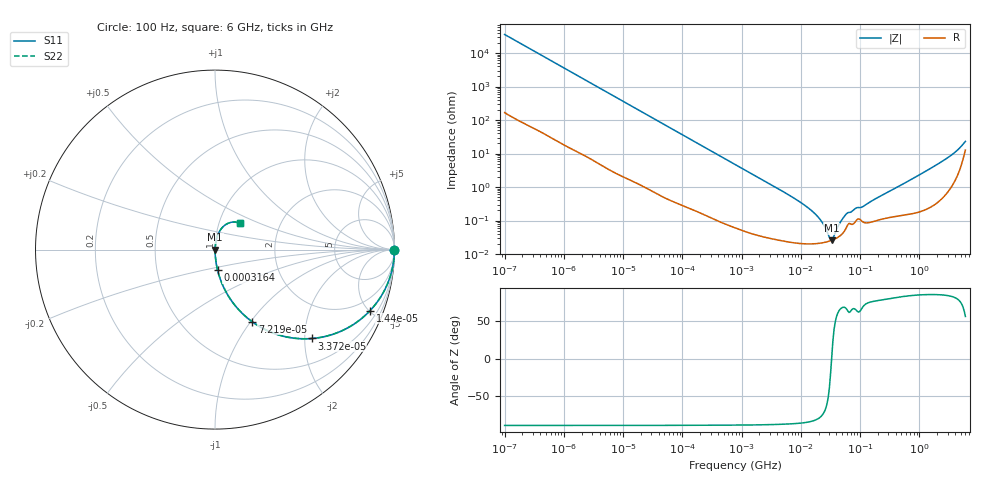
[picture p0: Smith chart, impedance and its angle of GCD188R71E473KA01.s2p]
!Murata Part Number: GCD188R71E473KA01
!These Parameters are Measured in Series Mode Connection
!Data Generated on Jan 08, 2026
!  o--ll--o
!Port1  Port2
!  o------o
!Operation Temp=25[degC], DC Bias Voltage=0[V]
!Freq. Start=100[Hz] Stop=6[GHz] 401[Steps]
# Hz S RI R 50
!Freq.(Hz) S11(Real) S11(Imag) S21(Real) S21(Imag) S12(Real) S12(Imag) S22(Real) S22(Imag)
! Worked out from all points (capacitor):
!   401 points, 100 Hz to 6 GHz, reference 50 ohm
!   read as one part in series: C = 44.3 nF near 109 Hz
!   lowest |Z| = 25.8 mohm at 33.3 MHz (marker M1)
!   series resonance near 33.08 MHz, so ESL is about 520 pH
!   S11 on the Smith chart (normalised r, x): 100 Hz: open; 14.4 kHz: 1.03, -5.06; 33.72 kHz: 1.01, -2.17; 72.19 kHz: 1.01, -1.02; 316.4 kHz: 1.00, -0.23; 6 GHz: 1.25, +0.38
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100  1 -0.00279  2.07e-05 0.00279  2.07e-05 0.00279  1 -0.00279
2008  0.9966 -0.0552  0.00336 0.0552  0.00336 0.0552  0.9966 -0.0552
5625  0.9759 -0.1508  0.0241 0.1508  0.0241 0.1508  0.9759 -0.1508
14402  0.8636 -0.3403  0.1364 0.3403  0.1364 0.3403  0.8636 -0.3403
33721  0.5405 -0.4952  0.4595 0.4952  0.4595 0.4952  0.5405 -0.4952
40335  0.4521 -0.4945  0.5479 0.4945  0.5479 0.4945  0.4521 -0.4945
72189  0.2069 -0.4016  0.7931 0.4016  0.7931 0.4016  0.2069 -0.4016
135116  0.0709 -0.2524  0.9291 0.2524  0.9291 0.2524  0.0709 -0.2524
316350  0.0146 -0.115  0.9854 0.115  0.9854 0.115  0.0146 -0.115
774597  0.00289 -0.0478  0.9971 0.0478  0.9971 0.0478  0.00289 -0.0478
6644369  0.000254 -0.00544  0.9997 0.00544  0.9997 0.00544  0.000254 -0.00544
1.555665e7  0.000204 -0.0019  0.9998 0.0019  0.9998 0.0019  0.000204 -0.0019
2.225763e7  0.000214 -0.000934  0.9998 0.000934  0.9998 0.000934  0.000214 -0.000934
3.045065e7  0.000243 -0.000191  0.9998 0.000191  0.9998 0.000191  0.000243 -0.000191
3.330331e7  0.000257 1.57e-05  0.9997 -1.57e-05  0.9997 -1.57e-05  0.000257 1.57e-05
3.64232e7  0.000275 0.000224  0.9997 -0.000224  0.9997 -0.000224  0.000275 0.000224
4.764863e7  0.000369 0.000884  0.9996 -0.000884  0.9996 -0.000884  0.000369 0.000884
5.960426e7  0.000653 0.00148  0.9993 -0.00148  0.9993 -0.00148  0.000653 0.00148
3.124326e8  0.00128 0.00732  0.9987 -0.00732  0.9987 -0.00732  0.00128 0.00732
2.34314e9  0.00735 0.0553  0.9927 -0.0553  0.9927 -0.0553  0.00735 0.0553
4.385646e9  0.0352 0.1166  0.9648 -0.1166  0.9648 -0.1166  0.0352 0.1166
6e9  0.1377 0.1472  0.8623 -0.1472  0.8623 -0.1472  0.1377 0.1472
